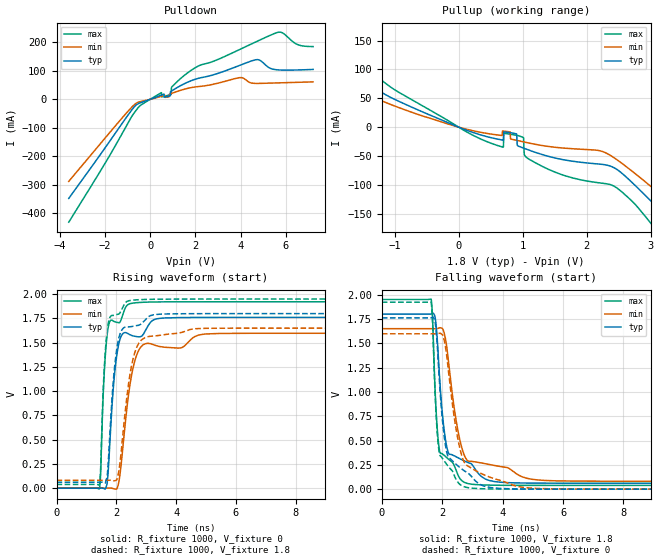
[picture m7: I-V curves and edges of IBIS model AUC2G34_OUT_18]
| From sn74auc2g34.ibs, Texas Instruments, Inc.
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[Model]   AUC2G34_OUT_18
Model_type  Output
Vref =   0
Rref =   1000
Cref =   30p
Vmeas =   0.9
| variable   typ   min   max
C_comp   6.70pF   0.45pF   21.41pF
| C_pullup   7.16pF   1.06pF   21.41pF
| C_pulldown   6.24pF   0.45pF   15.47pF
[Temperature Range]   40   100   -40
| Ambient temperature   25   85   -40
[Voltage range]   1.8   1.65   1.95
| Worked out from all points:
|   slope of the pulldown table from 0 to 0.27 V, typ, clamps not added: 34.4 ohm
|   slope of the pullup table from 0 to 0.27 V, typ, clamps not added: 24.7 ohm
|   rising waveform, R_fixture 1000, V_fixture 0: 20-80 % time 272ps typ, 402ps min, 178ps max; typ from 0 V to 1.76 V
|   falling waveform, R_fixture 1000, V_fixture 1.8: 20-80 % time 316ps typ, 480ps min, 196ps max; typ from 1.8 V to 0.061 V
|   rising waveform, R_fixture 1000, V_fixture 1.8: 20-80 % time 267ps typ, 393ps min, 176ps max; typ from 0.061 V to 1.8 V
|   falling waveform, R_fixture 1000, V_fixture 0: 20-80 % time 323ps typ, 489ps min, 196ps max; typ from 1.76 V to 0 V
[Pulldown]
| AUC2G34_OUT_18
|   Voltage   I(typ)   I(min)   I(max)
-3.6V     -348.1mA   -288.3mA   -431.6mA
-830mV    -38.96mA   -28.97mA   -62.23mA
-405mV    -11.33mA   -7.446mA   -19.55mA
495mV     14.95mA    10.62mA    23.51mA
885mV     12.29mA    19.09mA    15.87mA
925mV     28.57mA    20.19mA    16.9mA
960mV     30.15mA    21.18mA    44.34mA
2.04V     71.84mA    43.97mA    113.3mA
3.92V     118.2mA    75.86mA    173.7mA
4.62V     138.3mA    56mA       199.9mA
5.58V     103.9mA    57.61mA    233.8mA
7.2V      105mA      61.31mA    185.3mA
[Pullup]
| AUC2G34_OUT_18
|   Voltage   I(typ)   I(min)   I(max)
-3.6V     266.7mA    220.8mA    317.6mA
-2.61V    173.8mA    138mA      219.2mA
-2.13V    131.2mA    101.7mA    171.3mA
110mV     -4.812mA   -3.244mA   -7.318mA
695mV     -22.64mA   -6.828mA   -34.84mA
705mV     -8.169mA   -6.943mA   -10.57mA
975mV     -34.74mA   -24.57mA   -16.33mA
1.11V     -40.27mA   -27.85mA   -56.21mA
2.25V     -64.64mA   -42.33mA   -97.32mA
3.1V      -138.7mA   -111.5mA   -179.7mA
3.915V    -230.6mA   -188.2mA   -289.8mA
7.2V      -598.7mA   -504.1mA   -721.8mA
[Ramp]
| AUC2G34_OUT_18
| variable   typ   min   max
dV/dt_r   1.06/2.74E-10   0.96/4.06E-10   1.16/1.79E-10
dV/dt_f   1.05/3.18E-10   0.95/4.86E-10   1.15/1.97E-10
R_load = 1000
[Rising Waveform]
| AUC2G34_OUT_18
R_fixture =   1000
C_fixture =   0
L_fixture =   0
V_fixture =   0
V_fixture_min = 0
V_fixture_max = 0
|   Time   V(typ)   V(min)   V(max)
0s        7.645nV    26.05nV    1.116nV
1.43ns    61.14uV    -7.403uV   -6.788mV
1.595ns   -5.494mV   23.97uV    1.179V
1.72ns    139.6mV    660.4uV    1.643V
1.885ns   976.1mV    -3.183mV   1.726V
2.035ns   1.409V     6.135mV    1.709V
2.47ns    1.58V      1.093V     1.903V
2.91ns    1.59V      1.481V     1.917V
4.955ns   1.761V     1.589V     1.922V
22.2ns    1.761V     1.597V     1.922V
[Falling Waveform]
| AUC2G34_OUT_18
R_fixture =   1000
C_fixture =   0
L_fixture =   0
V_fixture =   1.8
V_fixture_min = 1.65
V_fixture_max = 1.95
|   Time   V(typ)   V(min)   V(max)
0s        1.8V       1.65V      1.95V
1.63ns    1.8V       1.65V      1.954V
1.68ns    1.808V     1.649V     1.749V
1.775ns   1.745V     1.649V     941mV
1.91ns    1.16V      1.659V     395.6mV
2.195ns   381.2mV    1.345V     312.1mV
2.515ns   324.1mV    609.2mV    149.1mV
2.825ns   277.5mV    297.1mV    59.61mV
4.225ns   66.5mV     211.4mV    39.47mV
22.2ns    61.07mV    81.21mV    38.69mV
[Rising Waveform]
| AUC2G34_OUT_18
R_fixture =   1000
C_fixture =   0
L_fixture =   0
V_fixture =   1.8
V_fixture_min = 1.65
V_fixture_max = 1.95
|   Time   V(typ)   V(min)   V(max)
0s        61.05mV    81.2mV     38.68mV
1.43ns    61.11mV    81.2mV     32.91mV
1.47ns    61.36mV    81.19mV    167.9mV
1.595ns   56.39mV    81.23mV    1.225V
1.715ns   199.3mV    81.77mV    1.675V
2.015ns   1.434V     85.98mV    1.79V
2.41ns    1.663V     1.077V     1.932V
2.855ns   1.7V       1.532V     1.945V
4.63ns    1.799V     1.644V     1.95V
22.2ns    1.8V       1.65V      1.95V
[Falling Waveform]
| AUC2G34_OUT_18
R_fixture =   1000
C_fixture =   0
L_fixture =   0
V_fixture =   0
V_fixture_min = 0
V_fixture_max = 0
|   Time   V(typ)   V(min)   V(max)
0s        1.761V     1.597V     1.922V
1.63ns    1.761V     1.597V     1.924V
1.68ns    1.768V     1.597V     1.71V
1.77ns    1.707V     1.597V     934mV
1.905ns   1.118V     1.603V     367mV
2.17ns    354.3mV    1.317V     246.4mV
2.47ns    252.3mV    596.1mV    93.89mV
2.76ns    182.7mV    260.4mV    21.65mV
5.135ns   867.8uV    7.321mV    190.3uV
22.2ns    24.86uV    4.493uV    10.93uV
